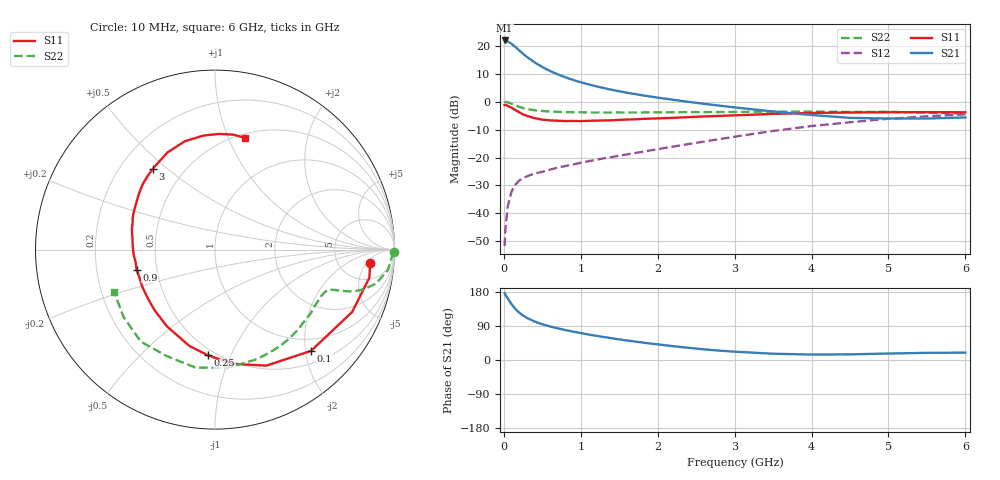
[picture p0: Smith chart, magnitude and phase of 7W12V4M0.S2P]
! Infineon Technologies  Discrete & RF Semiconductors
! BFS17W
! Si NPN RF Bipolar Junction Transistor in SOT323
! VCE = 12 V  IC = 4 mA
! Common Emitter S-Parameters:  August  1999
# GHz  S  MA  R  50
!  f  S11  S21  S12  S22
! GHz  MAG  ANG  MAG  ANG  MAG  ANG  MAG  ANG
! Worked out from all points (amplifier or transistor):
!   36 points, 10 MHz to 6 GHz, reference 50 ohm
!   highest |S21| = 21.9 dB at 10 MHz (marker M1)
!   |S21| within 3 dB of that: start of sweep to 177.5 MHz
!   unconditionally stable (mu >= 1): 675.1 MHz to 2.312 GHz; 5.325 GHz to end of sweep
!   at 250 MHz: K = 0.51, MSG = 22.2 dB, |S12| = -27.4 dB
!   at 1.4 GHz: K = 1.20, MAG = 9.3 dB, |S12| = -19.9 dB
!   at 6 GHz: K = 1.05, MAG = -1.9 dB, |S12| = -4.5 dB
!   S11 on the Smith chart (normalised r, x): 10 MHz: 10, -6; 100 MHz: 0.74, -2.11; 250 MHz: 0.46, -0.82; 900 MHz: 0.38, -0.11; 3 GHz: 0.34, +0.45; 6 GHz: 0.54, +1.15
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0.01  0.8679 -4.9  12.4 176.7  0.0026 77.7  0.9969 -0.9
0.02  0.8742 -10.3  12.35 172.6  0.0052 87.6  0.9842 -2.7
0.05  0.8397 -24.4  11.94 162.3  0.0133 78.2  0.9709 -6.7
0.1  0.7776 -46.5  10.79 147.3  0.0247 67.5  0.9171 -11.9
0.15  0.707 -66.1  9.478 134.5  0.0329 59.2  0.8568 -15.0
0.2  0.6443 -81.2  8.241 124.9  0.0388 55.1  0.8064 -16.8
0.25  0.5899 -93.9  7.165 117.3  0.0428 51.5  0.7667 -17.6
0.3  0.5554 -104.9  6.303 111.1  0.0462 51.0  0.7381 -18.1
0.4  0.5046 -122.0  5.028 101.5  0.0518 49.5  0.6998 -18.7
0.5  0.477 -134.9  4.156 94.3  0.0557 50.9  0.6789 -19.2
0.6  0.4617 -144.8  3.521 88.5  0.0608 52.0  0.6649 -20.0
0.7  0.4548 -153.0  3.074 83.5  0.066 54.0  0.6563 -21.2
0.9  0.4511 -165.7  2.438 74.9  0.0751 57.1  0.6452 -23.9
1.1  0.4534 -175.9  2.033 67.2  0.0859 60.1  0.6406 -27.2
1.3  0.4606 175.6  1.746 60.7  0.0968 62.9  0.6378 -31.0
1.6  0.4782 165.2  1.442 51.5  0.1138 66.1  0.6371 -36.9
2.2  0.5123 148.4  1.079 36.5  0.1567 71.5  0.6454 -50.5
3  0.568 127.7  0.788 22.0  0.2356 72.7  0.6529 -70.2
3.5  0.6024 116.2  0.666 16.6  0.2987 70.3  0.6628 -84.0
4.5  0.6386 95.8  0.512 14.9  0.427 59.0  0.6514 -114.3
5.5  0.6485 81.0  0.498 18.9  0.546 45.5  0.6331 -143.7
6  0.6445 75.2  0.521 19.3  0.5923 38.6  0.609 -156.9
